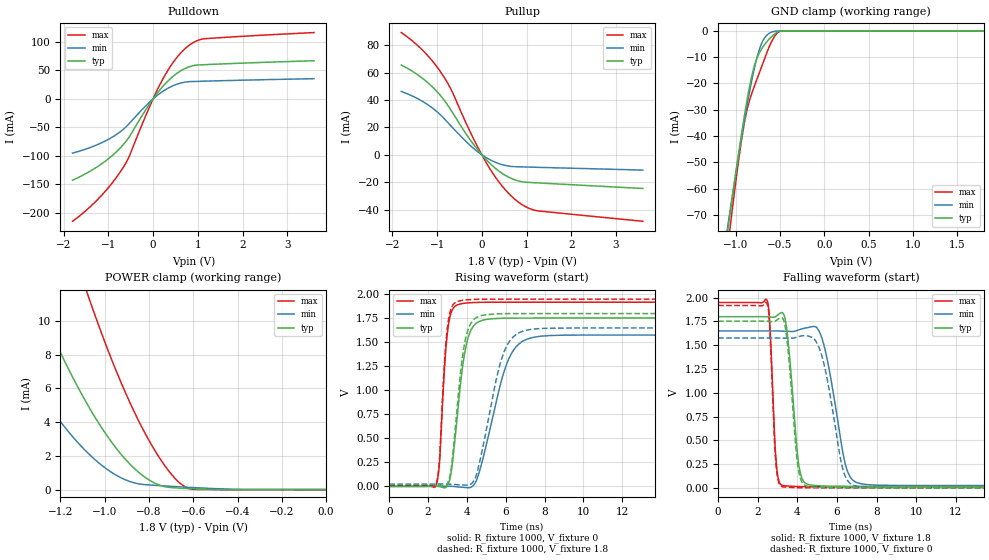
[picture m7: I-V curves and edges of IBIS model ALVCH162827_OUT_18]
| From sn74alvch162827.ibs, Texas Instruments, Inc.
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[Model]   ALVCH162827_OUT_18
Model_type  3-state
Enable   Active-Low
Vref =   0
Rref =   1000
Cref =   30p
Vmeas =   0.9
| variable   typ   min   max
C_comp   7.66pF   6.75pF   8.57pF
| C_pullup   8.76pF   7.27pF   9.47pF
| C_pulldown   12.36pF   9.13pF   16.14pF
| C_tri-state   7.66pF   6.75pF   8.57pF
[Temperature Range]   40   100   -40
| Ambient temperature   25   85   -40
[Voltage range]   1.8   1.65   1.95
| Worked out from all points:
|   slope of the pulldown table from 0 to 0.27 V, typ, clamps not added: 10.2 ohm
|   slope of the pullup table from 0 to 0.27 V, typ, clamps not added: 30.2 ohm
|   GND clamp passes 1 mA (typ) near -0.55 V on its own axis
|   POWER clamp passes 1 mA (typ) near -0.84 V on its own axis
|   rising waveform, R_fixture 1000, V_fixture 0: 20-80 % time 584ps typ, 1.17ns min, 336ps max; typ from 0 V to 1.75 V
|   falling waveform, R_fixture 1000, V_fixture 1.8: 20-80 % time 418ps typ, 785ps min, 240ps max; typ from 1.8 V to 0.016 V
|   rising waveform, R_fixture 1000, V_fixture 1.8: 20-80 % time 548ps typ, 1.02ns min, 326ps max; typ from 0.016 V to 1.8 V
|   falling waveform, R_fixture 1000, V_fixture 0: 20-80 % time 407ps typ, 780ps min, 235ps max; typ from 1.75 V to 0 V
[GND Clamp]
| ALVCH162827_OUT_18
|   Voltage   I(typ)   I(min)   I(max)
-1.8V     -267.3mA   -247.1mA   -300.4mA
-1.09V    -75.9mA    -74.07mA   -82.03mA
-1.075V   -72.18mA   -70.7mA    -77.81mA
-1.055V   -67.27mA   -66.24mA   -72.25mA
-920mV    -36.01mA   -37.55mA   -38.35mA
-875mV    -26.83mA   -28.78mA   -30.33mA
-820mV    -17.33mA   -18.99mA   -23.88mA
-775mV    -11.72mA   -12.1mA    -19.66mA
-720mV    -7.532mA   -5.789mA   -14.72mA
-615mV    -2.864mA   -799uA     -5.494mA
-485mV    -24.85uA   -61.55uA   -23.48uA
1.8V      60.47pA    9.416nA    28.01pA
[POWER Clamp]
| ALVCH162827_OUT_18
|   Voltage   I(typ)   I(min)   I(max)
-1.8V     29.67mA    18.6mA     47.93mA
-1.545V   19.46mA    11.49mA    33.45mA
-1.31V    11.36mA    6.08mA     21.55mA
-1.19V    7.854mA    3.858mA    16.15mA
-1.07V    4.862mA    2.091mA    11.3mA
-925mV    2.076mA    692.6uA    6.307mA
-850mV    1.061mA    349.7uA    4.157mA
-770mV    359.1uA    250.1uA    2.24mA
-695mV    116.6uA    189.9uA    848.9uA
-635mV    67.93uA    145.7uA    152.5uA
-585mV    37.09uA    111uA      9.499uA
-16.28fV  60.47pA    281.6pA    33.61pA
[Pulldown]
| ALVCH162827_OUT_18
|   Voltage   I(typ)   I(min)   I(max)
-1.8V     -142.5mA   -94.94mA   -214.6mA
-1.19V    -116mA     -78.24mA   -172.4mA
-925mV    -100.2mA   -67.56mA   -148.5mA
-690mV    -82.3mA    -54.81mA   -122.9mA
-535mV    -66.97mA   -43.32mA   -101mA
-105mV    -12.13mA   -7.634mA   -18.73mA
200mV     20.41mA    12.38mA    32.16mA
490mV     42.45mA    24.65mA    68.46mA
785mV     55.72mA    30.25mA    92.88mA
970mV     59.35mA    30.84mA    101.8mA
1.155V    60.2mA     31.26mA    105.7mA
3.6V      67.09mA    35.62mA    116.5mA
[Pullup]
| ALVCH162827_OUT_18
|   Voltage   I(typ)   I(min)   I(max)
-1.8V     65.54mA    46.25mA    89.25mA
-1.32V    55.67mA    38.89mA    76.19mA
-1.11V    49.72mA    34.29mA    68.65mA
-920mV    43.05mA    29.01mA    60.43mA
-685mV    32.34mA    20.89mA    47.55mA
-250mV    10.47mA    6.526mA    16.03mA
115mV     -4.131mA   -2.38mA    -6.642mA
450mV     -13.44mA   -7.131mA   -22.64mA
790mV     -18.81mA   -8.709mA   -33.84mA
1.02V     -20.1mA    -8.918mA   -38.54mA
1.25V     -20.5mA    -9.124mA   -40.92mA
3.6V      -24.58mA   -11.14mA   -48.53mA
[Ramp]
| ALVCH162827_OUT_18
| variable   typ   min   max
dV/dt_r   1.06/5.94E-10   0.95/1.18E-09   1.16/3.44E-10
dV/dt_f   1.10/4.35E-10   1.00/8.16E-10   1.18/2.54E-10
R_load = 1000
[Rising Waveform]
| ALVCH162827_OUT_18
R_fixture =   1000
C_fixture =   0
L_fixture =   0
V_fixture =   0
V_fixture_min = 0
V_fixture_max = 0
|   Time   V(typ)   V(min)   V(max)
0s        316.9pV    1.692nV    220.5pV
2.405ns   1.955mV    902.9uV    3.265mV
2.58ns    -2.06mV    1.576mV    225.4mV
2.85ns    -15.43mV   1.378mV    1.242V
3.03ns    21.36mV    1.198mV    1.652V
3.715ns   1.143V     -8.69mV    1.902V
4.48ns    1.698V     55.92mV    1.915V
6.105ns   1.752V     1.303V     1.918V
7.53ns    1.753V     1.556V     1.918V
50ns      1.753V     1.576V     1.918V
[Falling Waveform]
| ALVCH162827_OUT_18
R_fixture =   1000
C_fixture =   0
L_fixture =   0
V_fixture =   1.8
V_fixture_min = 1.65
V_fixture_max = 1.95
|   Time   V(typ)   V(min)   V(max)
0s        1.8V       1.65V      1.95V
2.5ns     1.799V     1.65V      1.96V
2.935ns   1.806V     1.65V      270.4mV
3.3ns     1.829V     1.648V     23.03mV
4.08ns    237.7mV    1.661V     13.53mV
4.62ns    32.01mV    1.69V      11.86mV
5.34ns    19.53mV    1.505V     11.27mV
6.5ns     16.41mV    194.6mV    11.11mV
7.24ns    16.08mV    41.69mV    11.09mV
50ns      15.91mV    23.52mV    11.08mV
[Rising Waveform]
| ALVCH162827_OUT_18
R_fixture =   1000
C_fixture =   0
L_fixture =   0
V_fixture =   1.8
V_fixture_min = 1.65
V_fixture_max = 1.95
|   Time   V(typ)   V(min)   V(max)
0s        15.91mV    23.52mV    11.08mV
2.405ns   17.23mV    24.46mV    15.66mV
2.58ns    13.02mV    24.84mV    249.8mV
2.845ns   1.556mV    24.09mV    1.286V
3.02ns    38.03mV    23.59mV    1.692V
3.685ns   1.206V     15mV       1.934V
4.395ns   1.745V     70.82mV    1.947V
5.865ns   1.798V     1.373V     1.95V
7.19ns    1.8V       1.631V     1.95V
50ns      1.8V       1.65V      1.95V
[Falling Waveform]
| ALVCH162827_OUT_18
R_fixture =   1000
C_fixture =   0
L_fixture =   0
V_fixture =   0
V_fixture_min = 0
V_fixture_max = 0
|   Time   V(typ)   V(min)   V(max)
0s        1.753V     1.576V     1.918V
2.5ns     1.752V     1.576V     1.922V
2.915ns   1.757V     1.576V     272.9mV
3.225ns   1.789V     1.574V     12mV
4.04ns    217.2mV    1.589V     2.253mV
4.53ns    14.94mV    1.597V     775uV
5.285ns   2.861mV    1.353V     167.6uV
6.355ns   396.1uV    158.8mV    21.75uV
7.04ns    128.5uV    14.76mV    6.437uV
50ns      -2.082nV   -2.095nV   -5.042nV
